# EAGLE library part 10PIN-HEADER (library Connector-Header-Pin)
10 pin Header Pin
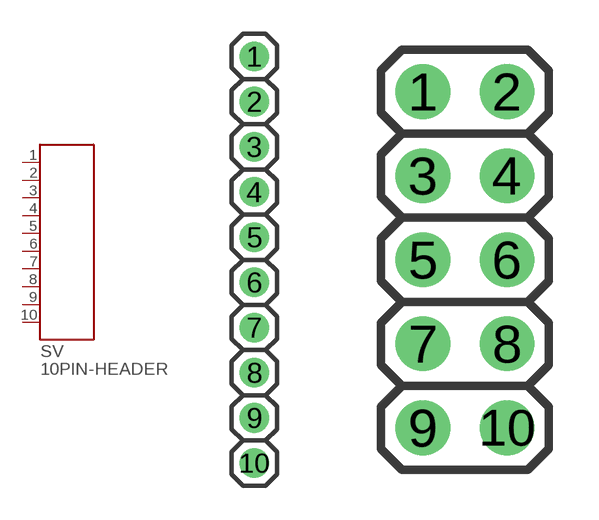
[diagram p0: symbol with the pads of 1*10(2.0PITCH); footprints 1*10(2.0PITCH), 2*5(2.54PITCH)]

Designator prefix SV

## 10PIN-HEADER-SINGLE_2PITCH  [1*10(2.0PITCH)]
1  1
2  2
3  3
4  4
5  5
6  6
7  7
8  8
9  9
10  10

## 10PIN-HEADER-DOUBLE_2.54PITCH  [2*5(2.54PITCH)]
Pads as for 1*10(2.0PITCH)

## 10PIN-HEADERSINGLE_2.54PITCH  [1*10(2.54PITCH)]
Pads as for 1*10(2.0PITCH)

## 10PIN-HEADERSINGLE-2PITCH_MOUNT  [NPPN101BFLD-RC]
Pads as for 1*10(2.0PITCH)

## 10PIN-HEADER  [XPPN101BFCN-RC]
Pads as for 1*10(2.0PITCH)

## Footprint 1*10(2.0PITCH) (pad centres in mm)
1 * 10 pin , 2.0 pitch Header Pin d0.8
drill 0.8: 1 0,9; 2 0,7; 3 0,5; 4 0,3; 5 0,1; 6 0,-1; 7 0,-3; 8 0,-5; 9 0,-7; 10 0,-9

## Footprint 2*5(2.54PITCH) (pad centres in mm)
2 * 5 pin Double Header Pin **male** (2.54mm pitch )
drill 1.1: 1 -1.27,3.81; 2 1.27,3.81; 3 -1.27,1.27; 4 1.27,1.27; 5 -1.27,-1.27; 6 1.27,-1.27; 7 -1.27,-3.81; 8 1.27,-3.81; 9 -1.27,-6.35; 10 1.27,-6.35

## Footprint 1*10(2.54PITCH) (pad centres in mm)
1 * 10 2.54mm pitch Header Pin d1.1
drill 1.1: 1 0,11.43; 2 0,8.89; 3 0,6.35; 4 0,3.81; 5 0,1.27; 6 0,-1.27; 7 0,-3.81; 8 0,-6.35; 9 0,-8.89; 10 0,-11.43

## Footprint NPPN101BFLD-RC (pad centres in mm)
NPPN101BFLD-RC 1*10 2.0mm pitch surface mount , D mounting style Store Infomation: Digi-Key http://dkc1.digikey.com/jp/digihome.html
smd 2.29 x 0.89: 1 -1.395,9; 2 1.395,7; 3 -1.395,5; 4 1.395,3; 5 -1.395,1; 6 1.395,-1; 7 -1.395,-3; 8 1.395,-5; 9 -1.395,-7; 10 1.395,-9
